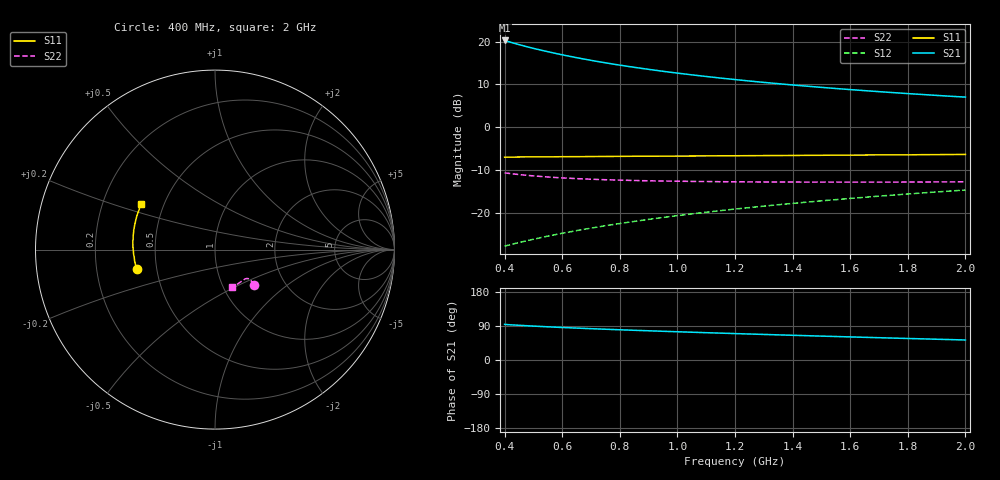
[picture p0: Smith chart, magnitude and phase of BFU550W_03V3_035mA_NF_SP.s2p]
! Filename:  P:\Prog\Test\Noise\ATS_data\Testdata_Net\06 Compressed Noise after Statistics\BFU550W_APM2013_11_D05_03p3V_035mA_NF_CM01_D.sf
! Date/Time: Tue 26/Mar/2013 16:25:21
! BFU550W_APM2013_11_D05_03p3V_1to35mA_NF_CM01_Bias9_R.sf
! Noise Parameter Data File
! BFU550W_APM2013_11_D05_03p3V_1to35mA_NF_CM01
! Date/time: Mon Mar 25 12:16:07 2013
! VAR V_out= 3.300000
! VAR I_out= 34.990000
! VAR V_in= 0.844400
! VAR I_in= 0.391900
! Device data file deembeded for feedlines and parallel
! Original file: \06 Compressed Noise after Statistics\BFU550W_APM2013_11_D05_03p3V_035mA_NF_CM01_R.sf
! Feed-files: PR019V01_070313_Feed1.s2p, PR019V01_070313_Feed2.s2p
! Parallel-file: PR019V01_070313_Par.s2p
# MHz S MA R 50
!  Freq-MHz  S11-mag  S11-arg  S21-mag  S21-arg  S12-mag  S12-arg  S22-mag  S22-arg
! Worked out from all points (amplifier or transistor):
!   37 points, 400 MHz to 2 GHz, reference 50 ohm
!   highest |S21| = 20.3 dB at 400 MHz (marker M1)
!   |S21| within 3 dB of that: start of sweep to 575.8 MHz
!   unconditionally stable (mu >= 1): 588.7 MHz to 1.835 GHz
!   at 500 MHz: K = 0.98, MSG = 22.3 dB, |S12| = -26.1 dB
!   at 1.1 GHz: K = 1.03, MAG = 14.8 dB, |S12| = -19.8 dB
!   at 2 GHz: K = 0.99, MSG = 10.8 dB, |S12| = -14.6 dB
!   lowest NFmin = 1.19 dB at 433 MHz
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400  0.448 -166.0  10.33 93.9  0.04102 69.9  0.2941 -42.0
433  0.4491 -168.2  9.581 92.3  0.04377 70.5  0.2853 -41.6
460  0.4509 -169.7  9.042 91.2  0.04605 70.9  0.2789 -41.4
500  0.4524 -172.0  8.349 89.5  0.04938 71.5  0.2711 -41.0
550  0.452 -174.4  7.635 87.6  0.05372 72.2  0.2633 -40.8
600  0.4543 -176.5  7.021 85.8  0.05797 72.6  0.2566 -40.6
650  0.4546 -178.5  6.5 84.2  0.06231 73.0  0.2522 -40.8
700  0.4561 179.7  6.052 82.6  0.06666 73.3  0.248 -41.0
750  0.4574 178.0  5.662 81.2  0.07103 73.5  0.2446 -41.3
800  0.4581 176.2  5.321 79.8  0.07543 73.7  0.2421 -41.9
850  0.4597 174.7  5.019 78.4  0.07978 73.8  0.2396 -42.2
900  0.4601 173.3  4.751 77.1  0.08426 73.9  0.2377 -42.8
950  0.4605 171.8  4.51 75.8  0.08872 73.9  0.2362 -43.5
1050  0.4627 169.2  4.099 73.3  0.09766 73.8  0.2338 -45.0
1150  0.4659 166.5  3.758 70.9  0.1066 73.6  0.2321 -46.7
1200  0.4658 165.4  3.612 69.7  0.1112 73.5  0.2314 -47.7
1250  0.4668 164.1  3.472 68.6  0.1157 73.3  0.2308 -48.4
1350  0.4687 161.9  3.231 66.3  0.1249 73.0  0.2298 -50.4
1500  0.4718 158.5  2.928 63.0  0.1387 72.2  0.2297 -53.7
1650  0.4752 155.2  2.681 59.9  0.1526 71.5  0.2296 -57.0
1750  0.4769 153.4  2.542 57.8  0.162 70.9  0.2293 -59.3
2000  0.483 148.2  2.253 52.8  0.1855 69.3  0.2311 -65.7
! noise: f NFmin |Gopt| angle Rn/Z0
400  1.194  0.4553  -170.3  0.059
460  1.199  0.4613  -168.3  0.0603
600  1.285  0.4611  -165.7  0.0626
800  1.292  0.4902  -161.1  0.0624
1000  1.331  0.5048  -156.6  0.0685
1200  1.424  0.5032  -153.4  0.08
1400  1.467  0.5238  -148  0.0899
1600  1.542  0.5292  -143.6  0.1092
1800  1.585  0.5282  -138.5  0.1415
2000  1.688  0.5354  -134.6  0.1668
